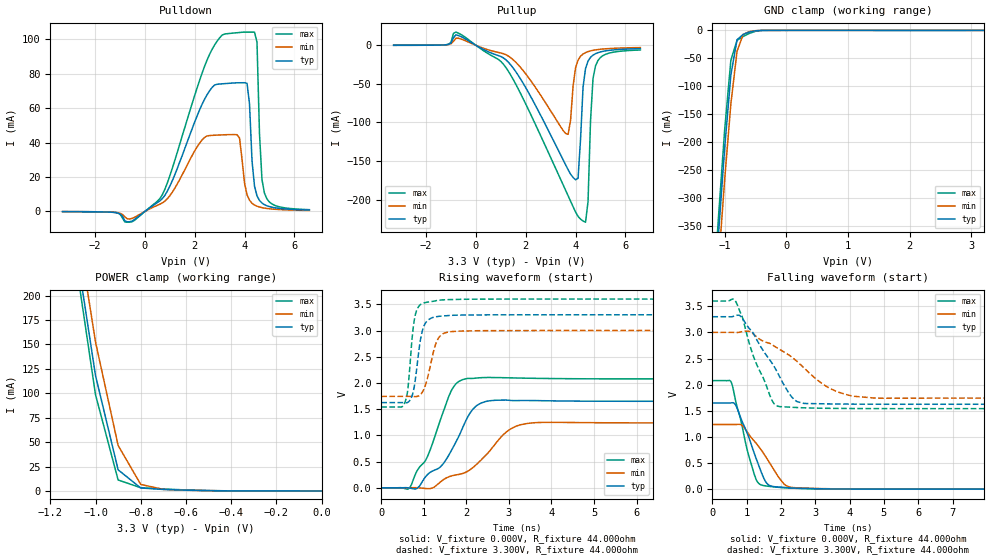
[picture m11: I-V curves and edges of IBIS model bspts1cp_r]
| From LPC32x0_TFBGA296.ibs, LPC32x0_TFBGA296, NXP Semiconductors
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| |   Rev 0.20 IBIS Model Design Automation Generation   |
| |   N O N - S I L I C O N   C O R R E L A T E D   |
| |   This IBIS [Model] is pre-Beta tactical support   |
| |  Note: this IBIS [Model] contains clamp curves generated   |
| |   through simulation which should not be relied upon   |
| bspts1cp
|   Bidirectional Pad 3v3
|   3state Output
|   Plain Input
|   1ns Slew Rate control
|   CMOS
|   Programmable between
|   - (p1=0, p2=1) plain input
|   - (p1=0, p2=0) with Pull Up
|   - (p1=1, p2=1) with Pull Down
|   - (p1=1, p2=0) with Repeater
|   Characterized at Core 1.2V and I/O 3.3V
| Repeater Mode (p1=1, p2=0)
[Model]   bspts1cp_r | of bspts1cp
Model_type   I/O
Polarity   Non-Inverting
Enable   Active-Low
|  Reciever Thresholds
Vinl   = 0.36V
Vinh   = 0.84V
| AC Test Load Conditions
Vref   = 0
Cref   = 1.2e-11
Rref   = 1000000000
Vmeas   = 0.6
| [Process Range]   typical   min   max
| C_comp edge width   400.000ps   400.000ps   400.000ps
| C_comp Tstrobe   40.000fs   40.000fs   40.000fs
C_comp   2.378pF   2.238pF   2.550pF
[Temperature Range]   25   125   -40
[Voltage Range]   3.30V   3.00V   3.60V
[GND Clamp Reference]   0.00V   0.00V   0.00V
[Pulldown Reference]   0.00V   0.00V   0.00V
[POWER Clamp Reference]   3.30V   3.00V   3.60V
[Pullup Reference]   3.30V   3.00V   3.60V
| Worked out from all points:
|   slope of the pulldown table from 0 to 0.495 V, typ, clamps not added: 97.1 ohm
|   slope of the pullup table from 0 to 0.495 V, typ, clamps not added: 59.3 ohm
|   GND clamp passes 1 mA (typ) near -0.51 V on its own axis
|   POWER clamp passes 1 mA (typ) near -0.63 V on its own axis
|   rising waveform, V_fixture 0.000V, R_fixture 44.000ohm: 20-80 % time 780ps typ, 1.07ns min, 628ps max; typ from 0 V to 1.65 V
|   falling waveform, V_fixture 0.000V, R_fixture 44.000ohm: 20-80 % time 570ps typ, 781ps min, 474ps max; typ from 1.65 V to 0 V
|   rising waveform, V_fixture 3.300V, R_fixture 44.000ohm: 20-80 % time 175ps typ, 230ps min, 140ps max; typ from 1.62 V to 3.3 V
|   falling waveform, V_fixture 3.300V, R_fixture 44.000ohm: 20-80 % time 910ps typ, 1.48ns min, 670ps max; typ from 3.3 V to 1.62 V
[GND Clamp]
| ref voltage   0.00V   0.00V   0.00V
|   Voltage   I(typ)   I(min)   I(max)
-3.3V     -4.198A    -4.223A    -4.188A
-1.2V     -526mA     -577.5mA   -497.2mA
-1.1V     -363.6mA   -417.9mA   -332.6mA
-1V       -210.1mA   -266.3mA   -177.3mA
-900mV    -79.71mA   -131.5mA   -53.29mA
-800mV    -16.76mA   -37.38mA   -17.81mA
-700mV    -7.164mA   -7.263mA   -10.92mA
-600mV    -3.002mA   -2.202mA   -5.445mA
-500mV    -699uA     -571.9uA   -1.612mA
-400mV    -79uA      -96.04uA   -163.6uA
3.2V      -4.082uA   6.375uA    -21.05uA
[Power Clamp]   | Vtable = Vcc - Vpad
| ref voltage   3.30V   3.00V   3.60V
|   Voltage   I(typ)   I(min)   I(max)
-3.3V     4.52A      4.504A     4.537A
-1.1V     269.9mA    299.6mA    255.3mA
-1V       118.1mA    152.4mA    98.46mA
-900mV    21.6mA     46.51mA    11.21mA
-800mV    3.019mA    6.665mA    3.25mA
-700mV    1.526mA    1.552mA    1.973mA
-600mV    767.7uA    705uA      1.011mA
-400mV    58.36uA    81.92uA    64.04uA
0V        755.1pA    5.591nA    627.9pA
[Pulldown]
| ref voltage   0.00V   0.00V   0.00V
|   Voltage   I(typ)   I(min)   I(max)
-3.3V     -80.68uA   -69.9uA    -74.32uA
-600mV    -5.92mA    -4.329mA   -6.172mA
500mV     5.147mA    3.568mA    5.922mA
2.5V      67.8mA     43.83mA    87.99mA
3.7V      74.65mA    44.53mA    103.7mA
4V        74.69mA    16.44mA    104.1mA
4.2V      62.38mA    6.514mA    104mA
4.3V      29.48mA    4.769mA    104mA
4.5V      9.068mA    3.068mA    98.17mA
4.6V      6.413mA    2.587mA    45.14mA
4.8V      3.956mA    1.96mA     10.6mA
6.6V      844.8uA    597.5uA    1.056mA
[Pullup]   | Vtable = Vcc - Vpad
| ref voltage   3.30V   3.00V   3.60V
|   Voltage   I(typ)   I(min)   I(max)
-3.3V     39.4uA     37.84uA    38.83uA
-800mV    13.66mA    9.123mA    17.15mA
1V        -14.52mA   -9.936mA   -20.86mA
3.7V      -161.3mA   -115.5mA   -195.1mA
4V        -174.4mA   -29.02mA   -216.2mA
4.1V      -172.4mA   -19.17mA   -221.9mA
4.4V      -30.01mA   -9.422mA   -229.4mA
4.5V      -20.39mA   -8.135mA   -202.5mA
4.6V      -15.6mA    -7.195mA   -97.92mA
4.7V      -12.75mA   -6.48mA    -42.98mA
4.8V      -10.87mA   -5.92mA    -26.67mA
6.6V      -4.278mA   -2.929mA   -6.056mA
[Ramp]
R_load   = 44.000ohm
|   dV/dt(typ)   dV/dt(min)   dV/dt(max)
dV/dt_r   1.003V/795.000ps   754.478mV/1.100ns   1.261V/635.000ps
dV/dt_f   1.021V/900.000ps   769.092mV/1.445ns   1.253V/655.000ps
[Rising Waveform]  | cubic spline decimation from 2001 points
V_fixture   = 0.000V
R_fixture   = 44.000ohm
|   Time   V(typ)   V(min)   V(max)
0s        20.64nV    394.3nV    10.69nV
655ps     -4.509mV   428.1uV    -8.81mV
1.09ns    255.6mV    -17.26mV   603.8mV
1.445ns   447.6mV    146.5mV    1.426V
1.67ns    745mV      230.7mV    1.89V
1.95ns    1.215V     283.3mV    2.072V
2.34ns    1.614V     524.7mV    2.1V
2.96ns    1.672V     1.078V     2.098V
3.43ns    1.665V     1.227V     2.09V
10ns      1.65V      1.237V     2.077V
[Falling Waveform]  | cubic spline decimation from 2001 points
V_fixture   = 0.000V
R_fixture   = 44.000ohm
|   Time   V(typ)   V(min)   V(max)
0s        1.65V      1.237V     2.077V
550ps     1.651V     1.237V     2.047V
680ps     1.607V     1.237V     1.685V
1.075ns   968.6mV    1.04V      607.6mV
1.275ns   589.2mV    879mV      186.7mV
1.43ns    318.4mV    745mV      79.84mV
1.665ns   71.21mV    507.4mV    52.77mV
2.08ns    33.15mV    105.1mV    27.9mV
2.31ns    23.85mV    34.24mV    19.69mV
10ns      523.6nV    1.302uV    543.1nV
[Rising Waveform]  | cubic spline decimation from 2001 points
V_fixture   = 3.300V
V_fixture_min = 3.000V
V_fixture_max = 3.600V
R_fixture   = 44.000ohm
|   Time   V(typ)   V(min)   V(max)
0s        1.625V     1.743V     1.541V
555ps     1.623V     1.743V     1.631V
625ps     1.631V     1.743V     1.892V
730ps     1.77V      1.742V     2.906V
785ps     1.982V     1.74V      3.244V
920ps     2.824V     1.778V     3.494V
1.005ns   3.092V     1.89V      3.527V
1.31ns    3.265V     2.805V     3.572V
1.58ns    3.286V     2.972V     3.589V
10ns      3.3V       3V         3.6V
[Falling Waveform]  | cubic spline decimation from 2001 points
V_fixture   = 3.300V
V_fixture_min = 3.000V
V_fixture_max = 3.600V
R_fixture   = 44.000ohm
|   Time   V(typ)   V(min)   V(max)
0s        3.3V       3V         3.6V
670ps     3.322V     2.999V     3.604V
840ps     3.3V       3.01V      3.346V
1.255ns   2.908V     2.935V     2.444V
1.725ns   2.425V     2.771V     1.718V
1.9ns     2.23V      2.698V     1.589V
2.47ns    1.675V     2.444V     1.562V
3.4ns     1.632V     1.936V     1.547V
4.135ns   1.627V     1.777V     1.543V
10ns      1.625V     1.743V     1.541V
